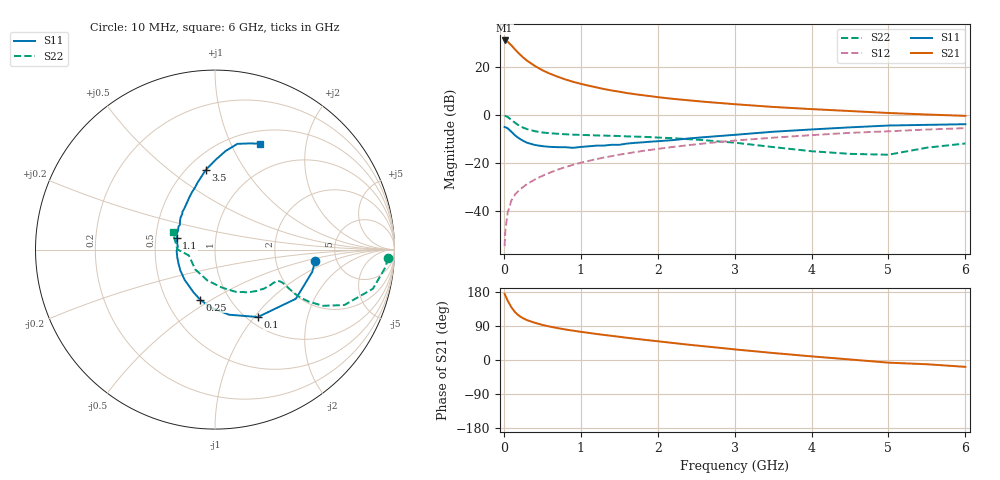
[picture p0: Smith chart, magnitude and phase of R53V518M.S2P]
! SIEMENS Small Signal Semiconductors
! BFR183
! Si NPN RF Bipolar Junction Transistor in SOT23
! VCE = 3.5 V  IC = 18 mA
! Common Emitter S-Parameters:  May  1996
# GHz  S  MA  R  50
!  f  S11  S21  S12  S22
! GHz  MAG  ANG  MAG  ANG  MAG  ANG  MAG  ANG
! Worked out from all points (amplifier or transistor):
!   36 points, 10 MHz to 6 GHz, reference 50 ohm
!   highest |S21| = 30.9 dB at 10 MHz (marker M1)
!   |S21| within 3 dB of that: start of sweep to 125.2 MHz
!   unconditionally stable (mu >= 1): 580.2 MHz to 2.366 GHz
!   at 250 MHz: K = 0.78, MSG = 26.9 dB, |S12| = -29.9 dB
!   at 1.4 GHz: K = 1.05, MAG = 12.3 dB, |S12| = -17.1 dB
!   at 6 GHz: K = 0.90, MSG = 2.6 dB, |S12| = -5.5 dB
!   S11 on the Smith chart (normalised r, x): 10 MHz: 3.43, -0.65; 100 MHz: 1.11, -1.04; 250 MHz: 0.73, -0.44; 1.1 GHz: 0.64, +0.09; 3.5 GHz: 0.61, +0.68; 6 GHz: 0.65, +1.30
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0.01  0.5614 -6.6  34.96 174.9  0.0019 86.3  0.9652 -2.7
0.02  0.5559 -12.9  34.74 169.9  0.0041 82.7  0.9554 -5.8
0.05  0.5273 -31.3  32.85 156.5  0.0094 77.6  0.9067 -13.9
0.1  0.4453 -57.5  27.41 138.5  0.0171 70.3  0.7842 -23.2
0.15  0.3717 -77.6  22.38 125.2  0.023 67.6  0.6782 -27.5
0.2  0.3258 -93.5  18.55 116.6  0.0275 67.4  0.5992 -29.0
0.25  0.2907 -106.7  15.58 110.1  0.032 67.5  0.5455 -29.3
0.3  0.2658 -117.0  13.39 105.3  0.0368 68.0  0.5084 -28.9
0.4  0.2386 -135.3  10.43 98.4  0.0455 69.7  0.4607 -27.6
0.5  0.2253 -149.0  8.45 92.6  0.0545 70.2  0.4323 -26.5
0.6  0.2176 -159.5  7.149 88.1  0.0636 70.7  0.417 -26.1
0.7  0.2145 -168.7  6.199 84.1  0.0732 70.5  0.4062 -26.0
0.8  0.214 -178.1  5.434 80.6  0.0827 70.0  0.3969 -26.3
0.9  0.208 175.8  4.863 77.4  0.0925 70.2  0.3896 -26.4
1.1  0.2231 163.2  4.046 71.7  0.1112 68.9  0.3805 -28.4
1.3  0.2313 153.0  3.448 66.2  0.1307 67.4  0.3724 -30.4
1.6  0.2545 139.9  2.841 58.6  0.1591 64.7  0.3586 -34.4
2.2  0.3007 121.9  2.151 44.9  0.2168 58.7  0.3289 -44.4
3.5  0.448 96.5  1.464 18.5  0.3373 42.6  0.2156 -79.5
4.5  0.5521 83.9  1.203 1.4  0.4254 29.9  0.1558 -134.9
5.5  0.6221 72.0  1.019 -11.2  0.4974 18.2  0.2094 179.8
6  0.6417 66.9  0.957 -18.1  0.5314 10.6  0.2558 157.2
